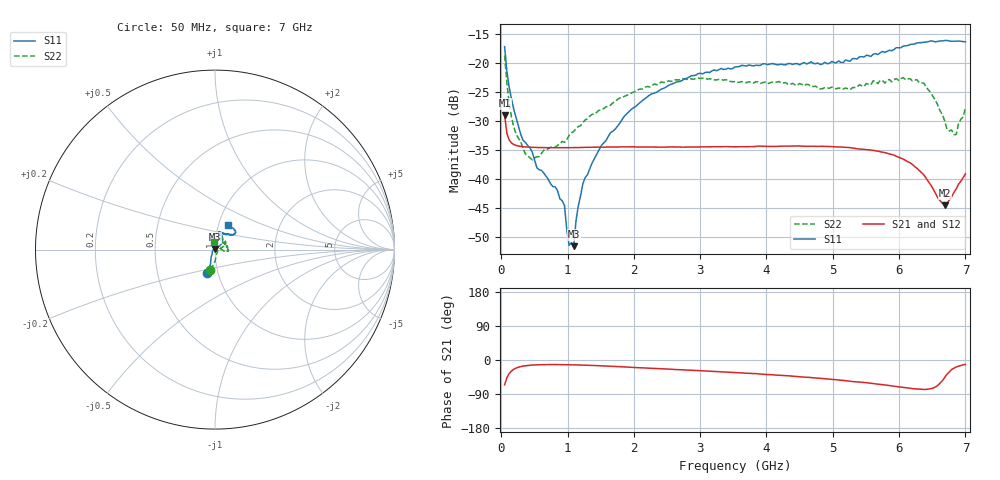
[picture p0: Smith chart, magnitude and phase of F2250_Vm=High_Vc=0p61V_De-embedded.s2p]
! Integrated Device Technology
! Corporate Headquarters
! 6024 Silver Creek Valley Road
! San Jose, CA 95138  USA
! Phone:  1-408-284-8200
! Toll Free:  1-800-223-1366
! Webpage:  http://www.idt.com/
! Timing and RF Division
! 515 Groton Road, Suite 102
! Westford, MA 01886-6024
! Device:  F2250
! Description: Voltage Variable RF Attenuator
! Frequency:  50.0 -  6000.00 MHz
! Package:  3x3 mm Thin QFN Plastic Package: 16 pin
! Ports:  2 RF, 3 DC
!  Pin  1  = GND
!  Pin  2  = NC
!  Pin  3  = RF1  = Port 1
!  Pin  4  = NC
!  Pin  5  = GND
!  Pin  6  = GND
!  Pin  7  = GND
!  Pin  8  = GND
!  Pin  9  = NC
!  Pin 10  = RF2  = Port 2
!  Pin 11  = NC
!  Pin 12  = GND
!  Pin 13  = GND
!  Pin 14  = VCNTRL
!  Pin 15  = VDD
!  Pin 16  = VMODE
! Vcntrl:  0.610 Volts
! Vmode:  +3.300 Volts
! Vdd:  +3.30  Volts
! Current:  1.278 mA
! Data:  The device was measured on a the F2250 evaluation board which has
!  individual transmission lines to the RF pins.  Data was collected
!  using a calibrated network analyzer.  The evaluation board was
!  de-embedded using a TRL calibration technique.
!  The reference plane is the edge of the package pin.
! Misc:  SN 10
!  Action Tracker AT0258
! Date Measured:  2014-11-26
! Date:  2015-10-15  MJV
! Note:
!  Integrated Device Technology supplies this data as a sample of measured
!  data at the package pin for this product.  Your particular data for this
!  product may vary.
!  Data was taken at 25 degrees C.
!  Integrated Device Technology reserves the right to change this data at anytime.
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# GHz S dB R 50
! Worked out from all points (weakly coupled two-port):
!   201 points, 50 MHz to 7 GHz, reference 50 ohm
!   highest |S21| = -28.98 dB at 50 MHz (marker M1); lowest = -44.5 dB at 6.687 GHz (marker M2)
!   lowest |S11| = -51.5 dB at 1.093 GHz (marker M3), VSWR 1.01, Z = 50 + j0.264 ohm
!   |S11| at or under -10 dB: start of sweep to end of sweep
!   |S22| runs from -36.7 to -18.7 dB; largest |S21 - S12| = 5e-05
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0.05  -17.17 -108.3  -28.98 -65.4  -28.98 -65.4  -18.71 -102.9
0.08475  -21.46 -107.2  -32.15 -46.6  -32.15 -46.6  -23.47 -90.1
0.15425  -26.23 -116.3  -33.77 -28.8  -33.77 -28.8  -29.36 -80.3
0.29325  -32.29 -126.8  -34.36 -17.4  -34.36 -17.4  -33.59 -51.8
0.36275  -33.67 -139.0  -34.45 -15.2  -34.45 -15.2  -35.64 -33.9
0.467  -35.36 -145.5  -34.51 -13.4  -34.52 -13.4  -36.67 -18.1
0.5365  -38.03 -153.9  -34.54 -12.7  -34.54 -12.7  -36.14 -11.9
0.9535  -44.55 171.5  -34.60 -12.3  -34.60 -12.3  -33.65 8.7
1.023  -51.39 138.5  -34.59 -12.5  -34.59 -12.5  -32.48 10.4
1.0925  -51.55 84.9  -34.58 -12.7  -34.57 -12.7  -31.77 12.2
1.12725  -47.14 58.3  -34.56 -12.9  -34.57 -12.9  -31.28 10.9
1.2315  -40.74 39.3  -34.53 -13.4  -34.54 -13.4  -30.24 9.9
1.6485  -31.99 40.6  -34.47 -16.5  -34.47 -16.5  -27.24 19.0
2.37825  -24.75 46.4  -34.46 -22.8  -34.47 -22.8  -23.56 28.7
3.525  -20.67 71.6  -34.43 -33.2  -34.43 -33.2  -23.21 56.7
4.7065  -20.07 71.9  -34.33 -46.9  -34.32 -46.9  -24.04 59.9
5.2625  -19.68 53.1  -34.57 -56.0  -34.56 -56.1  -24.55 36.8
5.85325  -17.80 40.5  -35.65 -67.4  -35.66 -67.5  -22.83 8.1
6.3745  -16.41 40.9  -39.30 -77.7  -39.31 -77.7  -23.47 -8.5
6.68725  -16.12 47.8  -44.54 -46.1  -44.53 -45.9  -29.94 11.9
6.861  -16.23 54.4  -41.70 -18.4  -41.66 -18.4  -32.33 60.8
7  -16.34 62.4  -39.08 -11.9  -39.05 -12.0  -27.75 97.8
